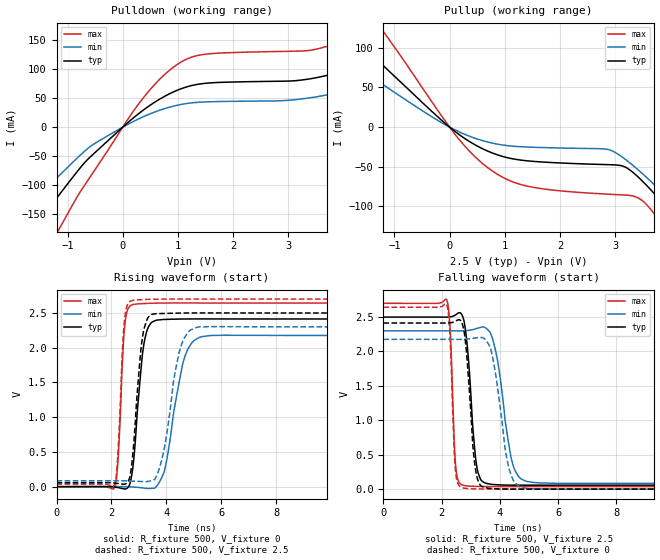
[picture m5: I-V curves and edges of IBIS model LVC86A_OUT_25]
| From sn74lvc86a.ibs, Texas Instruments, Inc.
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[Model]   LVC86A_OUT_25
Model_type  Output
Vref =   0
Rref =   500
Cref =   30p
Vmeas =   1.25
| variable   typ   min   max
C_comp   6.02pF   4.42pF   7.55pF
| C_pullup   5.82pF   4.42pF   6.92pF
| C_pulldown   6.21pF   4.42pF   7.55pF
[Temperature Range]   40   100   -40
| Ambient temperature   25   85   -40
[Voltage range]   2.5   2.3   2.7
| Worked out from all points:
|   slope of the pulldown table from 0 to 0.375 V, typ, clamps not added: 12.7 ohm
|   slope of the pullup table from 0 to 0.375 V, typ, clamps not added: 20 ohm
|   rising waveform, R_fixture 500, V_fixture 0: 20-80 % time 304ps typ, 546ps min, 182ps max; typ from 0 V to 2.41 V
|   falling waveform, R_fixture 500, V_fixture 2.5: 20-80 % time 249ps typ, 430ps min, 136ps max; typ from 2.5 V to 0.057 V
|   rising waveform, R_fixture 500, V_fixture 2.5: 20-80 % time 287ps typ, 513ps min, 181ps max; typ from 0.057 V to 2.5 V
|   falling waveform, R_fixture 500, V_fixture 0: 20-80 % time 241ps typ, 416ps min, 134ps max; typ from 2.41 V to 0 V
[Pulldown]
| LVC86A_OUT_25
|   Voltage   I(typ)   I(min)   I(max)
-5.5V     -598.1mA   -479.8mA   -766.5mA
-2.12V    -233mA     -174.4mA   -327.1mA
-1.575V   -168.1mA   -123.2mA   -244.7mA
-1.15V    -116.2mA   -83.21mA   -174.9mA
-565mV    -49.19mA   -31.72mA   -81.94mA
365mV     28.75mA    17.58mA    49.46mA
1.32V     73.05mA    42.4mA     122.5mA
4V        96.78mA    61.72mA    149.2mA
4.6V      117.3mA    77.78mA    177.9mA
5.77V     171.8mA    120.4mA    253.2mA
7.055V    245.3mA    179.5mA    351.5mA
11V       504.9mA    394.6mA    686.5mA
[Pullup]
| LVC86A_OUT_25
|   Voltage   I(typ)   I(min)   I(max)
-5.5V     363.4mA    279.9mA    508.8mA
-2.6V     169.4mA    122.6mA    251.6mA
-1.815V   117.7mA    83.03mA    179.1mA
-1.37V    88.47mA    61.37mA    136.9mA
170mV     -9.222mA   -5.867mA   -15.32mA
760mV     -32.2mA    -19.89mA   -54.58mA
2.905V    -47.35mA   -28.79mA   -84.65mA
3.45V     -65.04mA   -55.88mA   -90.57mA
3.92V     -100.7mA   -87.07mA   -129.3mA
4.19V     -123.8mA   -106.6mA   -157.6mA
4.495V    -151.4mA   -129.7mA   -191.8mA
11V       -830.2mA   -699.2mA   -1.022A
[Ramp]
| LVC86A_OUT_25
| variable   typ   min   max
dV/dt_r   1.47/3.24E-10   1.32/5.81E-10   1.61/1.89E-10
dV/dt_f   1.50/2.67E-10   1.37/4.56E-10   1.64/1.46E-10
R_load = 500
[Rising Waveform]
| LVC86A_OUT_25
R_fixture =   500
C_fixture =   0
L_fixture =   0
V_fixture =   0
V_fixture_min = 0
V_fixture_max = 0
|   Time   V(typ)   V(min)   V(max)
0s        177.7pV    3.876nV    17.91pV
2.145ns   -7.009mV   924.1uV    7.189mV
2.485ns   -33.44mV   345.3uV    2.315V
2.805ns   359.6mV    -5.848mV   2.624V
3.18ns    2.043V     -20.57mV   2.636V
3.65ns    2.397V     8.075mV    2.642V
3.97ns    2.407V     296.8mV    2.644V
4.64ns    2.414V     1.827V     2.644V
5.28ns    2.415V     2.159V     2.644V
24.99ns   2.414V     2.176V     2.644V
[Falling Waveform]
| LVC86A_OUT_25
R_fixture =   500
C_fixture =   0
L_fixture =   0
V_fixture =   2.5
V_fixture_min = 2.3
V_fixture_max = 2.7
|   Time   V(typ)   V(min)   V(max)
0s        2.5V       2.3V       2.7V
2.17ns    2.499V     2.3V       2.757V
2.3ns     2.503V     2.3V       2.276V
2.485ns   2.533V     2.299V     331.1mV
2.77ns    2.443V     2.301V     52.08mV
3.195ns   364.6mV    2.333V     38.86mV
3.58ns    77.95mV    2.32V      36.46mV
4.42ns    56.95mV    401.7mV    35.61mV
4.915ns   56.4mV     112.1mV    35.72mV
24.99ns   57.33mV    84.96mV    35.94mV
[Rising Waveform]
| LVC86A_OUT_25
R_fixture =   500
C_fixture =   0
L_fixture =   0
V_fixture =   2.5
V_fixture_min = 2.3
V_fixture_max = 2.7
|   Time   V(typ)   V(min)   V(max)
0s        57.33mV    84.96mV    35.94mV
2.14ns    50.92mV    85.64mV    53.44mV
2.465ns   35.85mV    84.79mV    2.352V
2.725ns   271.7mV    80.86mV    2.676V
3.115ns   2.104V     73.54mV    2.693V
3.51ns    2.486V     92.75mV    2.698V
3.915ns   2.493V     526.8mV    2.7V
4.51ns    2.499V     1.99V      2.7V
5.13ns    2.501V     2.295V     2.7V
24.99ns   2.5V       2.3V       2.7V
[Falling Waveform]
| LVC86A_OUT_25
R_fixture =   500
C_fixture =   0
L_fixture =   0
V_fixture =   0
V_fixture_min = 0
V_fixture_max = 0
|   Time   V(typ)   V(min)   V(max)
0s        2.414V     2.176V     2.644V
2.165ns   2.413V     2.176V     2.693V
2.29ns    2.417V     2.176V     2.208V
2.475ns   2.44V      2.176V     270.2mV
2.76ns    2.325V     2.178V     14.92mV
3.145ns   346.6mV    2.195V     2.729mV
3.48ns    20.42mV    2.182V     827.1uV
4.3ns     153.3uV    331.3mV    -330.9uV
4.72ns    -560.9uV   27.95mV    -270.1uV
24.99ns   -38.34nV   357.8pV    2.433nV
